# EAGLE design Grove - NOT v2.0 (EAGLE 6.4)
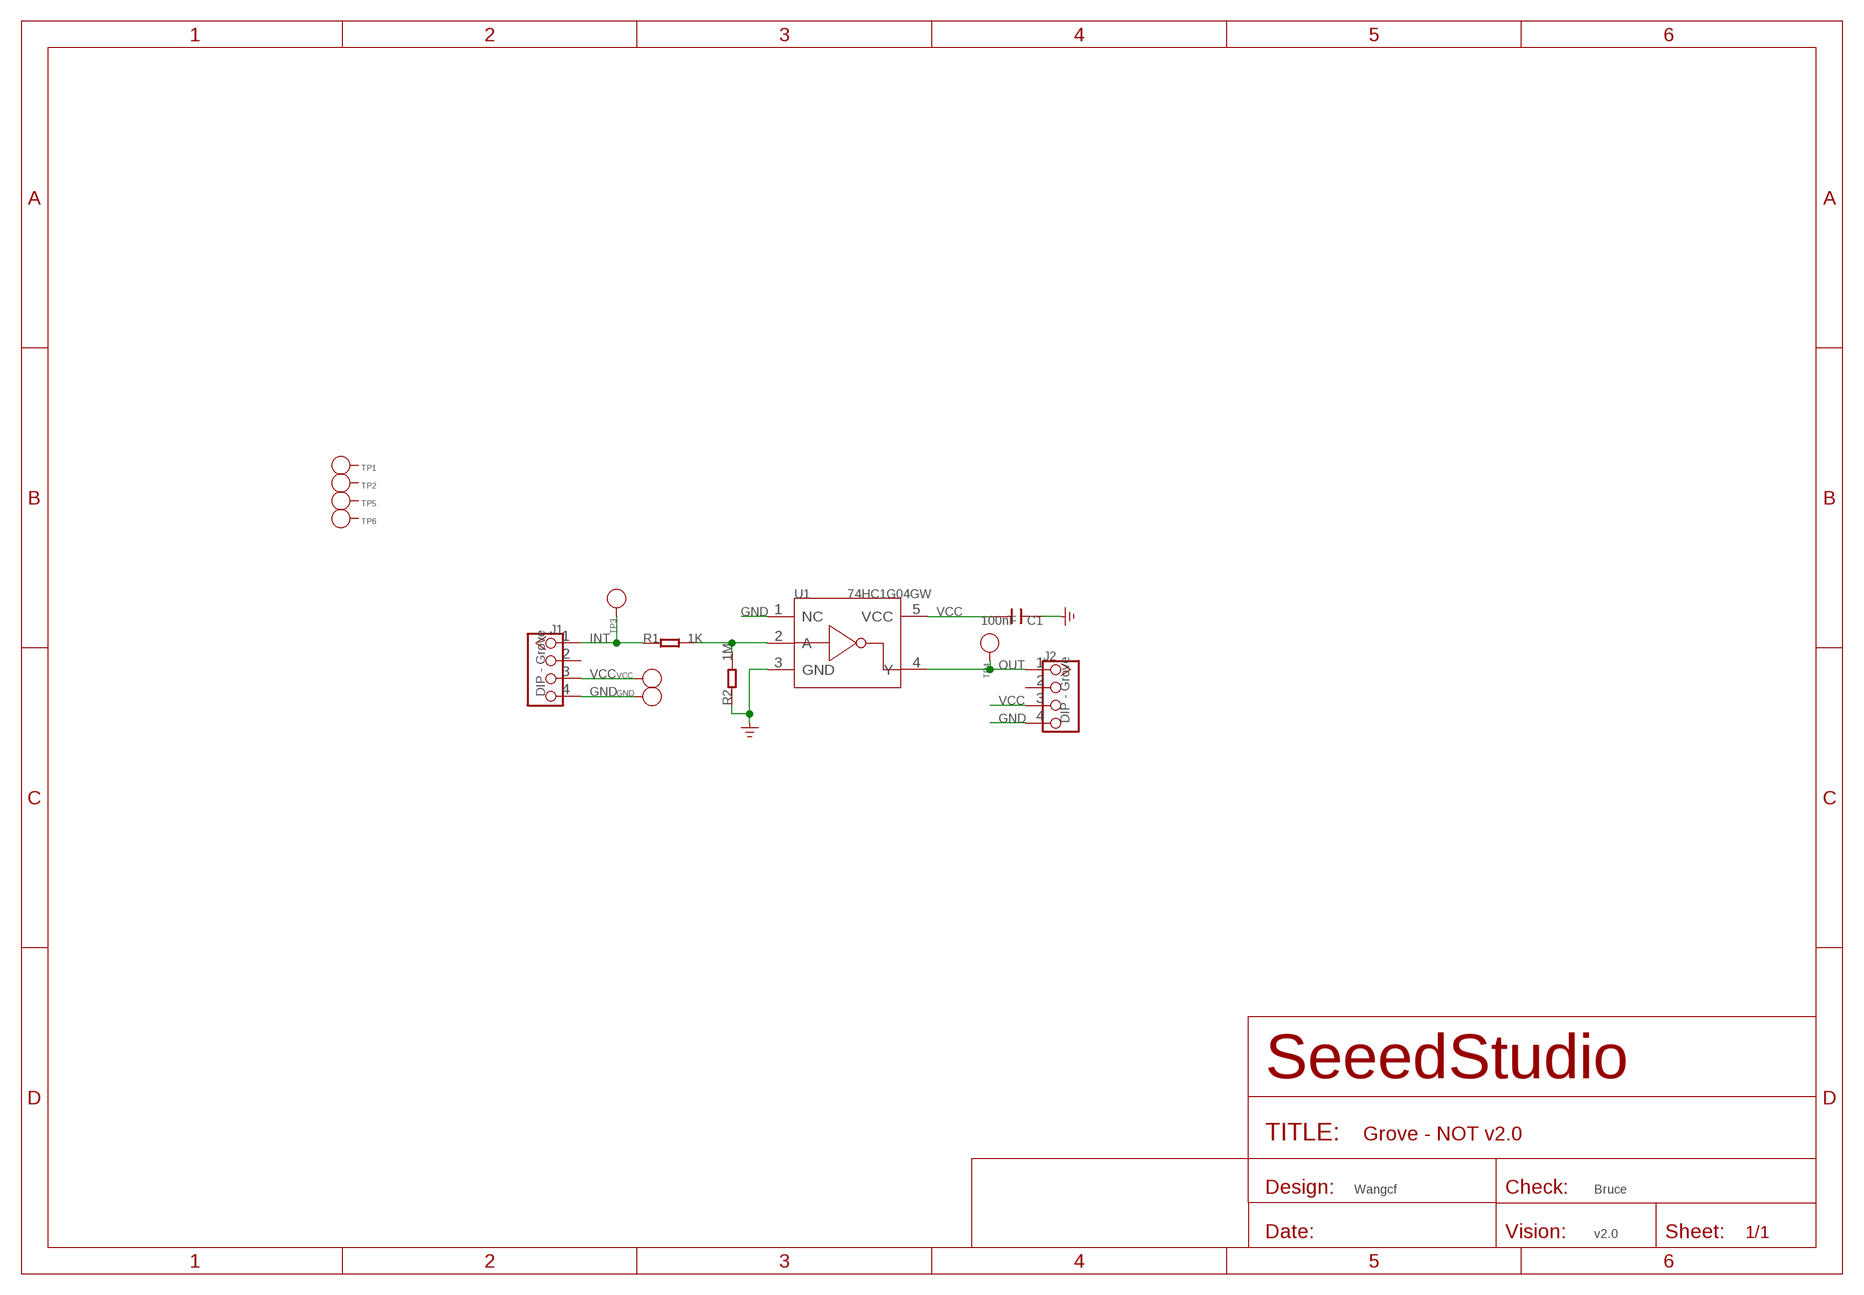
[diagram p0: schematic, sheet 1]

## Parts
C1  100nF  C-0603  [C0603]
GND  PAD-TEST-POINT'4545'  [TP_4545]
J1  DIP - Grove  TWIG-4P-2.0-2.0  [4P-2.0]
J2  DIP - Grove  TWIG-4P-2.0-2.0  [4P-2.0]
R1  1K  R-0603  [R0603]
R2  1M  R-0603  [R0603]
TP1  PAD-TEST-POINT'4545'  [TP_4545]
TP2  PAD-TEST-POINT'4545'  [TP_4545]
TP3  PAD-TEST-POINT'4545'  [TP_4545]
TP4  PAD-TEST-POINT'4545'  [TP_4545]
TP5  PAD-TEST-POINT'4545'  [TP_4545]
TP6  PAD-TEST-POINT'4545'  [TP_4545]
U1  74HC1G04GW  74HC1G04'GW'  [SOT-353]
VCC  PAD-TEST-POINT'4545'  [TP_4545]

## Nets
GND: C1.1 GND.T J1.4 J2.4 R2.1 U1.1(NC) U1.3(GND)
INT: J1.1 R1.1 TP3.T
N$4: R1.2 R2.2 U1.2(A)
OUT: J2.1 TP4.T U1.4(Y)
VCC: C1.2 J1.3 J2.3 U1.5(VCC) VCC.T
Unconnected: J1.2 J2.2 TP1.T TP2.T TP5.T TP6.T

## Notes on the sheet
- Wangcf | Bruce
- v2.0

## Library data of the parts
C1 = Discrete:C*: Ceramic Capacitors
GND TP1-TP6 VCC = Discrete:PAD-TEST-POINT; PARTNO: DNP
J1 J2 = Connector :TWIG-4P-2.0
R1 R2 = Discrete:R*
U1 = template:74HC1G04: 74HC1G04 and 74HCT1G04 are high-speed Si-gate CMOS devices. They provide an inverting buffer.

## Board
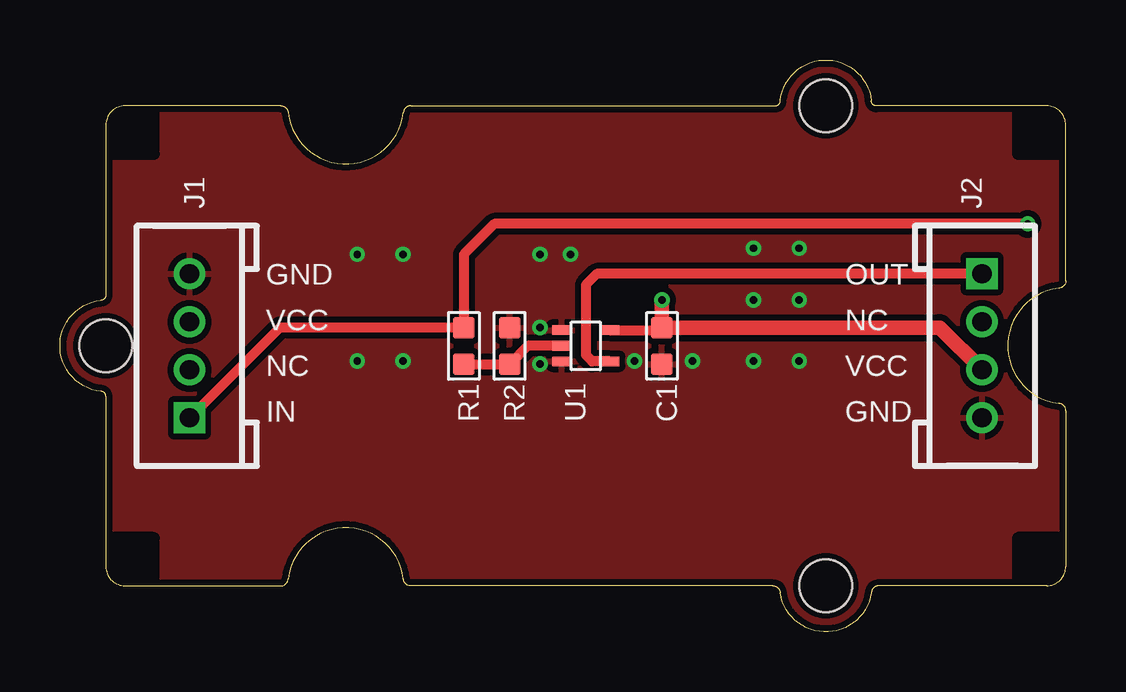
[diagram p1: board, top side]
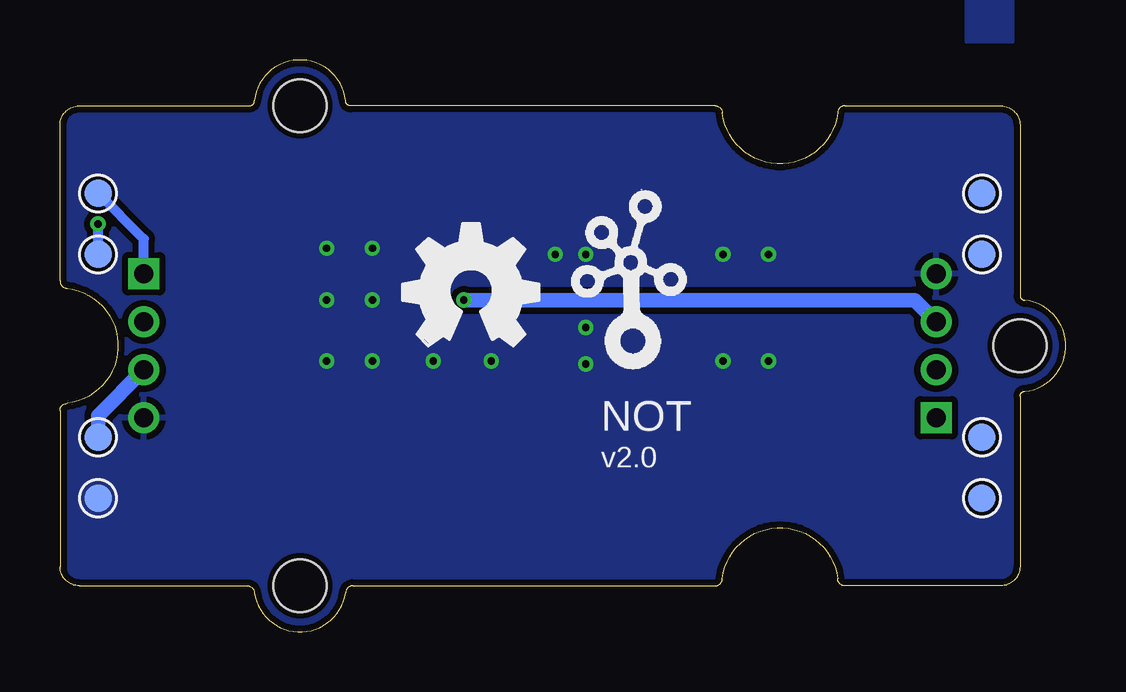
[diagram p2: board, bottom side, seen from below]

Size 41.91 x 23.83 mm. Coordinates in mm from the lower left corner, seen from the top.
Copper layers (1*16): Top 0.035mm / dielectric 1.5mm / Bottom 0.035mm
Design rules "SeeedStudio_DRU_no_angle_20130527 *": minimum track width 6mil, minimum drill 12mil, track to track 6mil, track to pad 6mil, pad to pad 6mil, via to via 6mil, smd to smd 0mil, copper to edge 10mil, drill to drill 10mil, minimum pad ring 10mil, minimum via ring 6mil, stop-mask expansion 2mil, vias tented up to drill 25mil, thermal gap 10mil

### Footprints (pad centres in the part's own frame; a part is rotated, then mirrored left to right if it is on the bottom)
C0603 = smd 0.889 x 0.889: 1 -0.762,0; 2 0.762,0
TP_4545 = smd 1.143 x 1.143: T 0,0
4P-2.0 = drill 0.8 pad 1.27 square: 1 -3,0 | drill 0.8 pad 1.27: 2 -1,0; 3 1,0; 4 3,0
R0603 = smd 0.889 x 0.889: 1 -0.762,0; 2 0.762,0
SOT-353 = smd 0.4 x 0.8: 1 -0.65,-1; 2 0,-1; 3 0.65,-1; 4 0.65,1; 5 -0.65,1
GROVE-2CONNECTOR = hole 2.2: -10,-10; -10,10; 20,0

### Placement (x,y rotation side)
C1  25.08,11.92 90 top
GND  40.32,5.57 0 bottom
J1  5.4,11.92 90 top
J2  38.42,11.92 270 top
R1  16.83,11.92 270 top
R2  18.73,11.92 270 top
TP1  3.49,18.27 0 bottom
TP2  3.49,15.73 0 bottom
TP3  40.32,15.73 0 bottom
TP4  40.32,18.27 0 bottom
TP5  3.49,8.11 0 bottom
TP6  3.49,5.57 0 bottom
U1  21.91,11.92 270 top
U$4  [TWIGLOGO]  18.1,11.92 0 bottom
U$5  [GROVE-2CONNECTOR]  21.91,11.92 180 top
U$6  [OSHW_FILLX200_NOTEXT]  27.62,11.92 0 bottom
VCC  40.32,8.11 0 bottom

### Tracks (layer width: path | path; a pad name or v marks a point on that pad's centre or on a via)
GND  (via drill 0.3 pad 0.64)
  other vias: 28.89,13.83 30.8,13.83 26.35,11.29 28.89,11.29 30.8,11.29 30.8,15.99 28.89,15.99 20,12.68 20,15.73 21.27,15.73 20,11.16 23.94,11.29 12.38,11.29 14.29,11.29 14.29,15.73 12.38,15.73
  pour Bottom: 2.22,26.53 4.13,26.53 4.13,24.62 2.22,24.62
  pour Bottom (isolate 0.254): -0.32,23.99 42.23,23.99 42.23,-0.14 -0.32,-0.14
  pour Top (isolate 0.254): -0.32,23.99 42.23,23.99 42.23,-0.14 -0.32,-0.14
INT  (via drill 0.3 pad 0.64)
  Top 0.406: v40.32,17 18.1,17 16.83,15.73 R1.1 9.16,12.68 J1.1
  Bottom 0.406: TP3.T v40.32,17
N$4
  Top 0.406: R1.2 R2.2 19.5,11.92 U1.2
OUT
  Top 0.406: U1.4 22.18,11.27 21.91,11.54 21.91,14.46 22.37,14.92 J2.1
  Bottom 0.406: J2.1 38.42,16.37 TP4.T
VCC  (via drill 0.3 pad 0.64)
  Top 0.406: U1.5 24.97,12.57 C1.2
  Top 0.61: J2.3 36.66,12.68 C1.2 v25.08,13.83
  Bottom 0.61: v25.08,13.83 6.3,13.83 J1.3 | VCC.T 40.32,9.02 J2.3

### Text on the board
tPlace: GND | OUT | VCC | NC | NC | VCC | IN | GND
bPlace: NOT | v2.0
